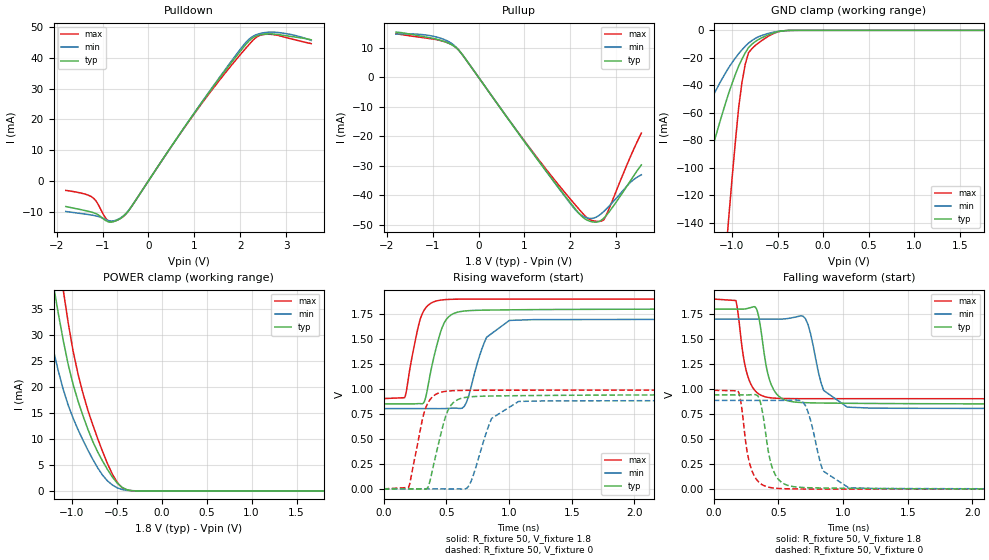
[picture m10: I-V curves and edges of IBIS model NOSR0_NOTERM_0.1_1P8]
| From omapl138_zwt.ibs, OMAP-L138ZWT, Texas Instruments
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|   Model Cell NOSR0_NOTERM_0.1_1P8
|NOSR0_NOTERM_0.1_1P8
[Model]   NOSR0_NOTERM_0.1_1P8
Model_type   3-state
Polarity   Non-Inverting
Enable   Active-Low
Cref =  15.0000pF
Rref =  100.0000M
Vref =  0V
Vmeas =  0.9
C_comp   3.009089p   2.23501p   3.95018p
[Temperature Range]   25   125   -40
[Voltage Range]   1.8   1.7   1.9
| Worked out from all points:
|   slope of the pulldown table from 0 to 0.27 V, typ, clamps not added: 44.1 ohm
|   slope of the pullup table from 0 to 0.27 V, typ, clamps not added: 45.3 ohm
|   GND clamp passes 1 mA (typ) near -0.50 V on its own axis
|   POWER clamp passes 1 mA (typ) near -0.46 V on its own axis
|   rising waveform, R_fixture 50, V_fixture 1.8: 20-80 % time 110ps typ, 134ps min, 95.7ps max; typ from 0.851 V to 1.8 V
|   rising waveform, R_fixture 50, V_fixture 0: 20-80 % time 113ps typ, 139ps min, 99.3ps max; typ from 0 V to 0.942 V
|   falling waveform, R_fixture 50, V_fixture 1.8: 20-80 % time 83.4ps typ, 98.5ps min, 76.6ps max; typ from 1.8 V to 0.851 V
|   falling waveform, R_fixture 50, V_fixture 0: 20-80 % time 81.1ps typ, 105ps min, 73.3ps max; typ from 0.942 V to 0 V
[POWER_clamp]
|   voltage   I(typ)   I(min)   I(max)
-1.8V     107.1mA    82.35mA    134.1mA
-1.327V   53.28mA    37.61mA    69.48mA
-1.182V   37.78mA    25.71mA    50.1mA
-1.091V   28.94mA    19.51mA    38.64mA
-1.073V   27.41mA    18.51mA    36.54mA
-981.8mV  20.5mA     14.01mA    26.92mA
-872.7mV  14.5mA     9.783mA    18.82mA
-709.1mV  7.513mA    4.449mA    10.09mA
-545.5mV  2.674mA    1.139mA    3.211mA
-436.4mV  654.9uA    255.5uA    594.1uA
-327.3mV  54.9uA     31.45uA    28.9uA
1.8V      5.504nA    121.3nA    1.604nA
[Pulldown]
|   voltage   I(typ)   I(min)   I(max)
-1.8V     -8.351mA   -9.956mA   -3.097mA
-1.2V     -10.35mA   -11.23mA   -5.575mA
-872.7mV  -13.35mA   -12.93mA   -13.07mA
-763.6mV  -13.31mA   -13.05mA   -13.22mA
-600mV    -12.16mA   -11.98mA   -12.14mA
-381.8mV  -8.669mA   -8.593mA   -8.643mA
1.145V    25.19mA    25.27mA    24.87mA
2.182V    45.44mA    46.03mA    44.25mA
2.345V    47.19mA    47.58mA    46.72mA
2.564V    47.83mA    48.35mA    47.74mA
3V        47.27mA    47.96mA    46.66mA
3.545V    45.94mA    45.74mA    44.7mA
[Pullup]
|   voltage   I(typ)   I(min)   I(max)
-1.8V     15.34mA    14.64mA    14.75mA
-981.8mV  13.15mA    13.91mA    12.94mA
-709.1mV  11.92mA    12.55mA    11.92mA
-490.9mV  10.05mA    10.24mA    10.12mA
1.145V    -24.96mA   -24.87mA   -24.59mA
2.018V    -42.87mA   -43.22mA   -41.64mA
2.236V    -46.95mA   -46.75mA   -45.58mA
2.455V    -48.93mA   -47.86mA   -48.45mA
2.618V    -48.93mA   -46.89mA   -48.85mA
2.727V    -47.76mA   -45.48mA   -48.34mA
3.273V    -35.91mA   -36.16mA   -28.15mA
3.545V    -29.71mA   -33.05mA   -18.91mA
[GND_clamp]
|   voltage   I(typ)   I(min)   I(max)
-1.8V     -229.3mA   -132mA     -818.5mA
-1.436V   -139.1mA   -79.12mA   -490.7mA
-1.073V   -53.39mA   -31.17mA   -167.2mA
-1.036V   -45.75mA   -27.16mA   -136.8mA
-927.3mV  -26.08mA   -17mA      -56.49mA
-890.9mV  -20.9mA    -14.21mA   -38.02mA
-854.5mV  -16.38mA   -11.64mA   -24.6mA
-818.2mV  -12.5mA    -9.275mA   -16.24mA
-709.1mV  -6.663mA   -4.641mA   -9.157mA
-527.3mV  -1.534mA   -1.158mA   -1.867mA
-381.8mV  -101.4uA   -119.7uA   -85.8uA
1.764V    4.755nA    203.2nA    1.222nA
[Ramp]
| variable   typ   min   max
dV/dt_f  0.5840345/83.79068p   0.5572725/99.27829p   0.6099212/76.90753p
dV/dt_r  0.5671716/0.1130405n  0.5337733/0.1375247n  0.5950157/99.4285p
R_load = 50
[Rising Waveform]
R_fixture = 50
V_fixture = 1.8
V_fixture_min = 1.7
V_fixture_max = 1.9
|   time   V(typ)   V(min)   V(max)
0s        851mV      803.4mV    903.9mV
167.2ps   851mV      803.4mV    912.7mV
270.4ps   852.8mV    803.4mV    1.592V
316.8ps   858mV      803.4mV    1.775V
455.2ps   1.574V     802.9mV    1.89V
517.6ps   1.722V     805.7mV    1.896V
642.4ps   1.78V      824.1mV    1.899V
820.8ps   1.79V      1.517V     1.9V
1.003ns   1.792V     1.686V     1.9V
5.21ns    1.8V       1.698V     1.9V
[Rising Waveform]
R_fixture = 50
V_fixture = 0
V_fixture_min = 0
V_fixture_max = 0
|   time   V(typ)   V(min)   V(max)
0s        84.48nV    277.7nV    33.22nV
199.2ps   48.86nV    347.5nV    13.56mV
307.2ps   -836.1uV   -523.8nV   683.5mV
345.6ps   2.676mV    1.624uV    841mV
500.8ps   749.2mV    -945.5uV   977.5mV
572.8ps   880.2mV    -433.9uV   984mV
680.8ps   920.3mV    31.71mV    986.5mV
861.6ps   929.6mV    705.8mV    987.4mV
1.077ns   933mV      875.4mV    987.8mV
6.031ns   942mV      885.5mV    988.3mV
[Falling Waveform]
R_fixture = 50
V_fixture = 1.8
V_fixture_min = 1.7
V_fixture_max = 1.9
|   time   V(typ)   V(min)   V(max)
0s        1.8V       1.7V       1.9V
170.4ps   1.8V       1.7V       1.886V
244ps     1.802V     1.7V       1.223V
321.6ps   1.82V      1.7V       981.1mV
426.4ps   1.113V     1.7V       915.6mV
525.6ps   907.4mV    1.7V       906.3mV
708ps     864.4mV    1.706V     904.5mV
850.4ps   860.7mV    986.1mV    904.3mV
1.032ns   858.3mV    820.3mV    904.2mV
5.22ns    851mV      805.1mV    903.9mV
[Falling Waveform]
R_fixture = 50
V_fixture = 0
V_fixture_min = 0
V_fixture_max = 0
|   time   V(typ)   V(min)   V(max)
0s        942mV      887.2mV    988.3mV
190.4ps   942mV      887.2mV    973.6mV
268.8ps   941.9mV    887.2mV    304.4mV
340.8ps   931.7mV    887.2mV    80.66mV
458.4ps   192.6mV    887.2mV    12.11mV
690.4ps   16.74mV    868.5mV    1.816mV
748ps     13.99mV    691mV      1.421mV
844.8ps   11.51mV    181.8mV    969.4uV
1.044ns   8.467mV    13.93mV    440.1uV
5.629ns   84.48uV    1.701mV    30.97nV
